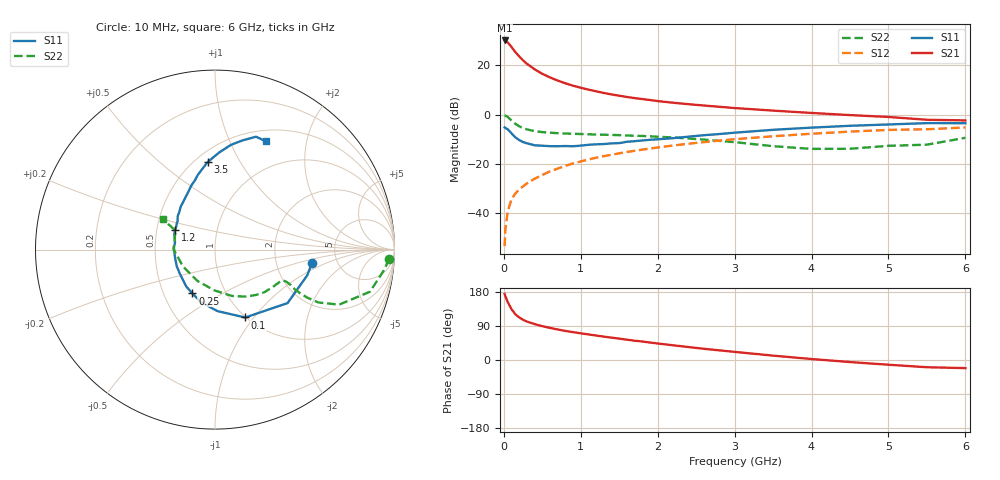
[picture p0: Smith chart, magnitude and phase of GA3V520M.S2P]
! Infineon Technologies  Discrete & RF Semiconductors
! BF775
! Si NPN RF Bipolar Junction Transistor in SOT23
! VCE = 3.5 V  IC = 20 mA
! Common Emitter S-Parameters:  May  1996
# GHz  S  MA  R  50
!  f  S11  S21  S12  S22
! GHz  MAG  ANG  MAG  ANG  MAG  ANG  MAG  ANG
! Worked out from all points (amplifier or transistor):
!   36 points, 10 MHz to 6 GHz, reference 50 ohm
!   highest |S21| = 30.1 dB at 10 MHz (marker M1)
!   |S21| within 3 dB of that: start of sweep to 107.8 MHz
!   unconditionally stable (mu >= 1): 387.9 MHz to 3.038 GHz
!   at 250 MHz: K = 0.87, MSG = 25.6 dB, |S12| = -29.2 dB
!   at 1.4 GHz: K = 1.12, MAG = 10.2 dB, |S12| = -16.4 dB
!   at 6 GHz: K = 0.95, MSG = 1.4 dB, |S12| = -5.3 dB
!   S11 on the Smith chart (normalised r, x): 10 MHz: 3.24, -0.68; 100 MHz: 0.99, -0.91; 250 MHz: 0.70, -0.37; 1.2 GHz: 0.62, +0.15; 3.5 GHz: 0.58, +0.74; 6 GHz: 0.63, +1.37
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0.01  0.5456 -7.8  32.17 174.2  0.0021 89.2  0.97 -3.0
0.02  0.5337 -15.6  31.7 168.4  0.0047 83.7  0.952 -6.5
0.05  0.5021 -36.4  29.47 153.2  0.0107 75.8  0.8949 -15.2
0.1  0.4141 -66.0  23.62 134.0  0.0189 69.9  0.7567 -23.9
0.15  0.3426 -87.9  18.69 120.6  0.0248 66.3  0.6466 -27.1
0.2  0.3031 -104.9  15.21 112.2  0.03 66.6  0.5768 -27.5
0.25  0.2749 -117.3  12.64 106.1  0.0346 66.6  0.5296 -27.1
0.3  0.2603 -128.2  10.78 101.4  0.0397 67.4  0.4984 -26.5
0.4  0.2372 -145.8  8.34 94.8  0.0494 69.2  0.4606 -24.9
0.5  0.2322 -156.9  6.738 89.2  0.059 70.2  0.4393 -24.3
0.6  0.2274 -167.3  5.692 84.7  0.0698 70.2  0.4275 -24.2
0.7  0.2268 -176.3  4.922 80.5  0.0795 70.2  0.4178 -24.5
0.8  0.2287 176.8  4.315 76.8  0.0907 69.7  0.4109 -25.1
0.9  0.2264 170.2  3.863 73.5  0.1011 69.3  0.406 -25.8
1.1  0.2426 159.4  3.215 67.5  0.1216 68.1  0.3972 -28.3
1.2  0.248 153.3  2.974 64.5  0.1323 67.2  0.3922 -29.4
1.6  0.2795 138.0  2.279 53.6  0.1731 63.3  0.3746 -35.9
2.2  0.3306 120.5  1.74 38.8  0.2344 56.9  0.3413 -47.7
3.5  0.4894 94.8  1.202 11.5  0.3615 40.5  0.2273 -90.9
4.5  0.5906 81.3  0.975 -5.4  0.4501 26.9  0.2014 -152.3
5.5  0.6693 70.0  0.783 -19.1  0.5022 11.9  0.244 154.3
6  0.6664 64.9  0.76 -21.4  0.5458 7.6  0.3365 149.8
